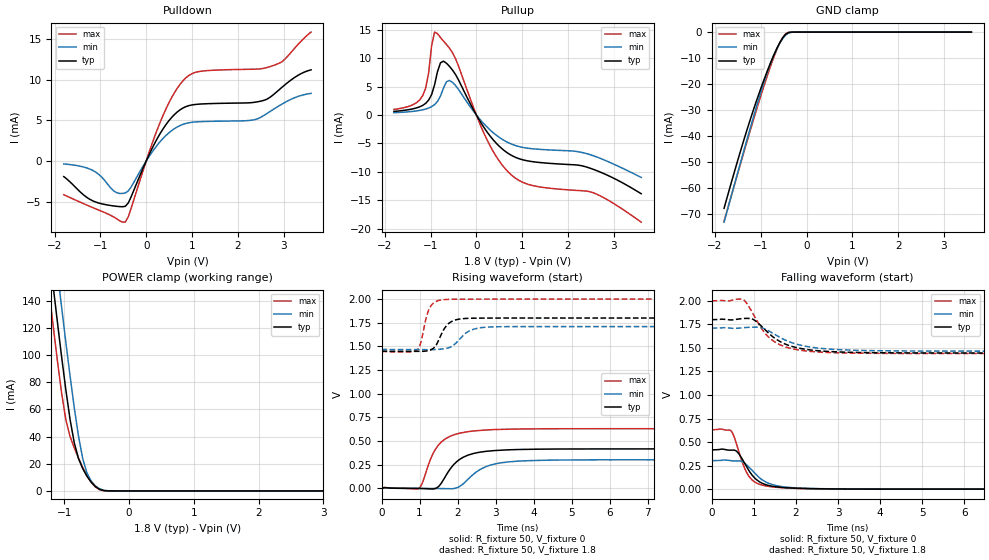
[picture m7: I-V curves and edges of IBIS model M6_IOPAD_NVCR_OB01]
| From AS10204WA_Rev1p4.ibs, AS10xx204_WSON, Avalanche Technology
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[Model] M6_IOPAD_NVCR_OB01
Model_type I/O
Enable   Active-High
Vinl  =  0.54
Vinh  =  1.26
Vmeas =  0.9
Cref  =  30e-12
| Capacitance  typ   min   max
C_comp   3.869840e-12   3.575244e-12   4.208825e-12
| Variables   typ   min   max
[GND Clamp Reference]   0   0   0
[POWER Clamp Reference]   1.8   1.71   2
[Pulldown Reference]   0   0   0
[Pullup Reference]   1.8   1.71   2
[Temperature Range]   25   105   -40
[Voltage Range]   1.8   1.71   2
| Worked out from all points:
|   slope of the pulldown table from 0 to 0.27 V, typ, clamps not added: 88.4 ohm
|   slope of the pullup table from 0 to 0.27 V, typ, clamps not added: 80.1 ohm
|   GND clamp passes 1 mA (typ) near -0.46 V on its own axis
|   POWER clamp passes 1 mA (typ) near -0.44 V on its own axis
|   falling waveform, R_fixture 50, V_fixture 0: 20-80 % time 409ps typ, 493ps min, 329ps max; typ from 0.417 V to 0 V
|   falling waveform, R_fixture 50, V_fixture 1.8: 20-80 % time 714ps typ, 842ps min, 588ps max; typ from 1.8 V to 1.45 V
|   rising waveform, R_fixture 50, V_fixture 0: 20-80 % time 559ps typ, 653ps min, 484ps max; typ from 0 V to 0.417 V
|   rising waveform, R_fixture 50, V_fixture 1.8: 20-80 % time 291ps typ, 400ps min, 205ps max; typ from 1.45 V to 1.8 V
[GND Clamp]
| Voltage   I(typ)   I(min)   I(max)
-1.8V     -67.84mA   -73.19mA   -72.81mA
-1.499V   -49.26mA   -53.93mA   -54.28mA
-1.303V   -37.87mA   -41.64mA   -42.4mA
-1.108V   -27.29mA   -29.68mA   -30.84mA
-912.4mV  -17.6mA    -18.46mA   -19.84mA
-782.1mV  -11.7mA    -11.87mA   -13.01mA
-651.7mV  -6.447mA   -6.494mA   -6.896mA
-521.4mV  -2.255mA   -2.526mA   -2.141mA
-456.2mV  -849.3uA   -1.156mA   -679.4uA
-391mV    -172uA     -356.5uA   -88.88uA
-260.7mV  -2.088uA   -12.98uA   -254.3nA
3.6V      0A         0A         0A
[POWER Clamp]
| Voltage   I(typ)   I(min)   I(max)
-1.8V     419.8mA    456.6mA    390.9mA
-1.238V   178mA      215.7mA    148.4mA
-1.173V   151mA      188.6mA    121.7mA
-1.108V   124.5mA    161.8mA    96mA
-1.043V   98.85mA    135.4mA    72.14mA
-977.6mV  74.56mA    109.6mA    52.56mA
-912.4mV  52.76mA    84.78mA    40.16mA
-847.2mV  35.48mA    61.36mA    31.71mA
-716.9mV  16.42mA    23.91mA    17.31mA
-651.7mV  10.9mA     13.27mA    11.28mA
-456.2mV  1.168mA    1.554mA    921.1uA
3.6V      0A         0A         0A
[Pulldown]
| Voltage   I(typ)   I(min)   I(max)
-1.8V     -1.924mA   -361uA     -4.159mA
-1.173V   -4.896mA   -1.141mA   -5.734mA
-716.9mV  -5.541mA   -3.657mA   -6.882mA
-456.2mV  -5.586mA   -3.936mA   -7.526mA
-391mV    -5.174mA   -3.688mA   -6.878mA
310.3mV   3.446mA    2.431mA    4.855mA
558.6mV   5.391mA    3.762mA    7.858mA
806.9mV   6.547mA    4.532mA    9.919mA
1.179V    7.023mA    4.851mA    11.06mA
2.352V    7.231mA    5.076mA    11.32mA
2.834V    8.456mA    6.576mA    11.9mA
3.6V      11.24mA    8.341mA    15.9mA
[Pullup]
| Voltage   I(typ)   I(min)   I(max)
-1.8V     628.3uA    396.4uA    967.2uA
-1.173V   1.677mA    903.2uA    3.367mA
-1.043V   2.6mA      1.212mA    7.324mA
-977.6mV  3.564mA    1.459mA    12.11mA
-912.4mV  5.287mA    1.824mA    14.55mA
-782.1mV  9.175mA    3.345mA    13.58mA
-651.7mV  9.08mA     5.842mA    12.38mA
-456.2mV  7.117mA    5.186mA    9.904mA
248.3mV   -3.143mA   -2.237mA   -4.604mA
744.8mV   -6.991mA   -5.033mA   -10.39mA
2.559V    -9.556mA   -7.166mA   -13.67mA
3.6V      -13.83mA   -10.96mA   -18.82mA
[Ramp]
dV/dt_r   0.25025/0.55882n  0.181396/0.652512n  0.378271/0.483969n
dV/dt_f   0.212589/0.713715n  0.146939/0.84212n  0.335614/0.588184n
R_load = 50
[Falling Waveform]
R_fixture = 50
V_fixture = 0
V_fixture_min = 0
V_fixture_max = 0
| Time   V(typ)   V(min)   V(max)
0s        417.1mV    302.3mV    630.5mV
463.6ps   414.7mV    301.2mV    617.4mV
530.2ps   414.8mV    300.4mV    558.9mV
607ps     395.5mV    301mV      453.7mV
789.6ps   268.3mV    273mV      214.1mV
994.9ps   130.2mV    181.9mV    84.28mV
1.334ns   40.92mV    65.23mV    30.5mV
1.728ns   16.33mV    23.24mV    13.57mV
3.783ns   611.4uV    961.3uV    578.2uV
21.88ns   104.5nV    449.1nV    135.6nV
[Falling Waveform]
R_fixture = 50
V_fixture = 1.8
V_fixture_min = 1.71
V_fixture_max = 2
| Time   V(typ)   V(min)   V(max)
0s        1.8V       1.71V      2V
734.6ps   1.812V     1.714V     2.017V
834.5ps   1.814V     1.718V     1.973V
990.2ps   1.802V     1.72V      1.855V
1.229ns   1.71V      1.708V     1.676V
1.448ns   1.619V     1.656V     1.578V
1.883ns   1.519V     1.558V     1.493V
2.543ns   1.469V     1.497V     1.456V
5.298ns   1.446V     1.466V     1.441V
21.88ns   1.446V     1.465V     1.441V
[Rising Waveform]
R_fixture = 50
V_fixture = 0
V_fixture_min = 0
V_fixture_max = 0
| Time   V(typ)   V(min)   V(max)
0s        58.89nV    367.7nV    108.9nV
967.4ps   -441.9uV   -264.5uV   -3.638mV
1.074ns   -1.686mV   -374.3uV   57.27mV
1.349ns   -6.571mV   -792.5uV   362.9mV
1.583ns   61.13mV    -2.726mV   493.5mV
2.013ns   293.6mV    10.71mV    578.7mV
2.666ns   386.6mV    214.6mV    614.9mV
3.353ns   407.2mV    280.1mV    625.5mV
4.675ns   415.7mV    299.2mV    629.9mV
21.88ns   417.1mV    302.3mV    630.5mV
[Rising Waveform]
R_fixture = 50
V_fixture = 1.8
V_fixture_min = 1.71
V_fixture_max = 2
| Time   V(typ)   V(min)   V(max)
0s        1.446V     1.465V     1.441V
944.3ps   1.447V     1.465V     1.466V
1.021ns   1.447V     1.465V     1.524V
1.268ns   1.459V     1.465V     1.907V
1.438ns   1.514V     1.467V     1.976V
1.644ns   1.683V     1.474V     1.994V
2.009ns   1.786V     1.557V     1.999V
2.375ns   1.798V     1.675V     1.999V
2.913ns   1.799V     1.706V     1.999V
21.88ns   1.8V       1.71V      2V
